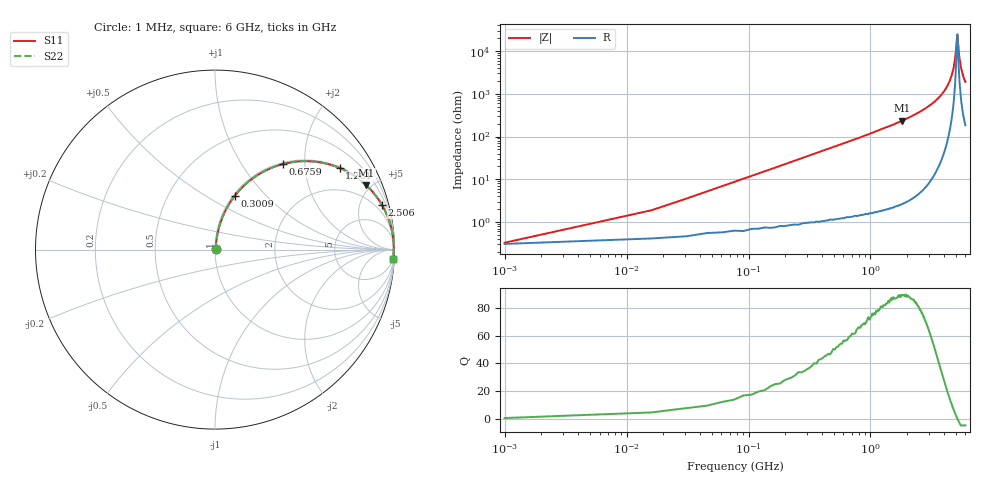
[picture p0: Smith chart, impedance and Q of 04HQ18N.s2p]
! Coilcraft 0403HQ-18N Chip Inductor
! 13 February 2004
# MHZ S MA R 50
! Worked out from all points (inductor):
!   401 points, 1 MHz to 6 GHz, reference 50 ohm
!   read as one part in series: L = 18 nH near 31 MHz
!   highest Q = 89.5 at 1.816 GHz (marker M1), where L = 20.5 nH
!   self-resonance near 5.145 GHz
!   S11 on the Smith chart (normalised r, x): 1 MHz: 1.01, +0.00; 300.9 MHz: 1.02, +0.68; 675.9 MHz: 1.03, +1.56; 1.261 GHz: 1.04, +3.03; 2.506 GHz: 1.08, +7.43; 6 GHz: 4, -38
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1  0.003301 19.9  0.997 -0.1  0.997 -0.1  0.003301 19.9
45.993  0.052 81.2  0.993 -3.0  0.993 -3.0  0.052 81.2
90.985  0.102 80.6  0.989 -5.8  0.989 -5.8  0.102 80.6
180.97  0.199 76.3  0.972 -11.5  0.972 -11.5  0.199 76.3
300.95  0.321 69.7  0.938 -18.7  0.938 -18.7  0.321 69.7
675.887  0.609 51.5  0.783 -37.5  0.783 -37.5  0.609 51.5
1005.832  0.759 39.9  0.641 -49.3  0.641 -49.3  0.759 39.9
1260.79  0.83 33.2  0.547 -56.1  0.547 -56.1  0.83 33.2
1815.697  0.916 23.0  0.391 -66.4  0.391 -66.4  0.916 23.0
2010.665  0.934 20.4  0.348 -69.0  0.348 -69.0  0.934 20.4
2505.582  0.963 15.0  0.259 -74.3  0.259 -74.3  0.963 15.0
3000.5  0.979 11.0  0.191 -78.1  0.191 -78.1  0.979 11.0
4005.332  0.993 5.0  0.087 -82.9  0.087 -82.9  0.993 5.0
4620.23  0.996 2.1  0.038 -82.4  0.038 -82.4  0.996 2.1
4815.198  0.996 1.3  0.024 -79.6  0.024 -79.6  0.996 1.3
5010.165  0.996 0.6  0.01 -67.5  0.01 -67.5  0.996 0.6
5115.148  0.996 0.1  0.004751 -32.5  0.004751 -32.5  0.996 0.1
5160.14  0.996 -0.0  0.004067 6.0  0.004067 6.0  0.996 -0.0
5355.108  0.996 -0.8  0.014 71.3  0.014 71.3  0.996 -0.8
5505.083  0.995 -1.3  0.023 77.6  0.023 77.6  0.995 -1.3
5700.05  0.995 -2.0  0.035 80.3  0.035 80.3  0.995 -2.0
6000  0.994 -3.0  0.052 81.5  0.052 81.5  0.994 -3.0
